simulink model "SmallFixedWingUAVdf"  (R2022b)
settings: Solver=ode4  StartTime=0  StopTime=stoptime  FixedStep=0.001  RelTol=1e-3  EnableMultiTasking=on
PreLoadFcn:
  | asbswarm_vehicledata; % load in workspace variables
PostLoadFcn:
  | open_system([gcs,'/MATLAB Animation Display/MATLAB',10,'Animation']);
InitFcn:
  | InitDatactrl
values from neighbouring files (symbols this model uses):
  env = struct    [InitDatactrl.m]
  F = Fattr + Frep    [APF.m]
  q = ix-1    [bspline_deboor.m]
  SenorSampleTime = 0.01    [InitDatactrl.m]
  sensors = struct    [InitDatactrl.m]
  uav = struct    [InitDatactrl.m]    (also in InitDatactrldf.m)
undefined symbols (not defined in the file or in its folder): Busy, Continuous, DiscIntNeverNeededParam, Dryden, Earth, Light, MIL, Newton, pa28, r, Raphson, sigbuilder_block, Wait, WGS84
libraries: simulink x37, aerolibactuator x10, sharedtransform x6, aerolibatmos2 x4, aerolibasang x4, aerolibwind2 x4, aerolibtransform2 x3, aerolibconvert2 x3, aerolibfltsims x2, shared6dof x2, aerolibnav x2, aerolibanimutils x1
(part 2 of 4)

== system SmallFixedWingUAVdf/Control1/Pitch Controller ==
  Pitch cmd : Inport
  Pitch act : Inport  Port=2
  pqr : Inport  Port=3
  Add1 : Sum  Inputs=+-
  Add6 : Sum  Inputs=+-
  Gain2 : Gain  Gain=-1
  PID_Pitch : Subsystem
  PID_PitchRate : Subsystem
  Selector : Selector  InputPortWidth=3  IndexOptions=Index vector (dialog)  Indices=2  OutputSizes=1
  elevatorCmd : Outport  VectorParamsAs1DForOutWhenUnconnected=off
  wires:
  PID_PitchRate/1(y) -> Gain2/1  "elevatorCmd"
  [reset] -> PID_PitchRate/2(reset_i)
  [reset] -> PID_Pitch/2(reset_i)
  Add1/1 -> PID_Pitch/1(e_theta)
  Add6/1 -> PID_PitchRate/1(x)
  Pitch act/1 -> Add1/2
  Gain2/1 -> elevatorCmd/1
  Selector/1 -> Add6/2  "q"
  PID_Pitch/1(qCmd) -> Add6/1
  pqr/1 -> Selector/1
  Pitch cmd/1 -> Add1/1

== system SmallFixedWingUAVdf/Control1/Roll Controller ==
  Roll cmd : Inport
  Roll act : Inport  Port=2
  pqr : Inport  Port=3
  Add2 : Sum  Inputs=+-
  Add3 : Sum  Inputs=+-
  PID_Roll : Subsystem
  PID_RollRate : Subsystem
  Selector1 : Selector  InputPortWidth=3  IndexOptions=Index vector (dialog)  Indices=1  OutputSizes=1
  aileronCmd : Outport  VectorParamsAs1DForOutWhenUnconnected=off
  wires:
  PID_RollRate/1(y) -> aileronCmd/1  "aileronCmd"
  Add2/1 -> PID_Roll/1(x)
  Add3/1 -> PID_RollRate/1(x)
  Selector1/1 -> Add3/2
  [reset] -> PID_RollRate/2(reset_i)
  [reset] -> PID_Roll/2(reset_i)
  pqr/1 -> Selector1/1
  Roll act/1 -> Add2/2
  PID_Roll/1(y) -> Add3/1
  Roll cmd/1 -> Add2/1

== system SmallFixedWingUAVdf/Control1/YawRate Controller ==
  psi_dot Cmd : Inport
  psi_dot : Inport  Port=2
  <YawRateCmd> : Inport  Port=3
  Add4 : Sum  Inputs=+-
  PID_YawRate : Subsystem
  Sum2 : Sum  Inputs=++|
  rudderCmd : Outport  VectorParamsAs1DForOutWhenUnconnected=off
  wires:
  Sum2/1 -> rudderCmd/1  "rudderCmd"
  Add4/1 -> PID_YawRate/1(x)
  [reset] -> PID_YawRate/2(reset_i)
  PID_YawRate/1(y) -> Sum2/2
  psi_dot/1 -> Add4/2
  psi_dot Cmd/1 -> Add4/1

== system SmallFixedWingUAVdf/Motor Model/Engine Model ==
  dt : Inport
  Airspeed : Inport  Port=2
  Constant4 : Constant  Value=0
  Get To : Subsystem
  Mass Conversion : aerolibconvert2/Mass Conversion  IU=lbm  OU=kg
  Mux : Mux  Inputs=2
  Mux1 : Mux  Inputs=3
  Thrust Available (lbs) : Fcn  Expr=u(1) - 0.047*sqrt(u(1))*u(2)
  kg2N : Gain  Gain=env.ISA_g  SaturateOnIntegerOverflow=on
  Thrust_b : Outport  Unit=kg*m/s^2  VectorParamsAs1DForOutWhenUnconnected=off
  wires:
  kg2N/1 -> Mux1/1
  Constant4/1 -> Mux1/3, Mux1/2
  Mass Conversion/1 -> kg2N/1
  Mux1/1 -> Thrust_b/1
  Airspeed/1 -> Mux/2
  Thrust Available (lbs)/1 -> Mass Conversion/1
  Mux/1 -> Thrust Available (lbs)/1
  Get To/1(To) -> Mux/1
  dt/1 -> Get To/1(dt)

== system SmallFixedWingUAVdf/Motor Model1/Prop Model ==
  dt : Inport
  Airspeed : Inport  Port=2
  Constant : Constant  Value=uav.prop.Ct
  Constant1 : Constant  Value=env.ISA_rho0
  Constant2 : Constant  Value=uav.prop.Dp
  Constant3 : Constant  Value=uav.prop.decay
  Constant4 : Constant  Value=0
  Constant5 : Constant  Value=uav.prop.Kv
  Constant6 : Constant  Value=uav.prop.U
  Mux : Mux  Inputs=3
  Mux1 : Mux  Inputs=3
  Product : Product  Inputs=4
  Product1 : Product  Inputs=3
  Saturation : Saturate  UpperLimit=1.0  LowerLimit=0
  Saturation1 : Saturate  UpperLimit=inf  LowerLimit=0
  Square : Math  Operator=square
  Square1 : Math  Operator=square
  Square2 : Math  Operator=square
  decay : Fcn  Expr=u(1)-u(3)*abs(u(2))/sqrt(u(1))
  min->s : Gain  Gain=1/60
  Thrust_b : Outport  Unit=kg*m/s^2  VectorParamsAs1DForOutWhenUnconnected=off
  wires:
  Constant4/1 -> Mux1/2, Mux1/3
  Product/1 -> Mux/1  "T0"
  Mux1/1 -> Thrust_b/1
  dt/1 -> Saturation/1
  Product1/1 -> min->s/1  "N"
  Airspeed/1 -> Mux/2  "Airspeed"
  Constant/1 -> Product/1
  min->s/1 -> Square/1
  Constant1/1 -> Product/2
  Constant2/1 -> Square2/1
  Square1/1 -> Product/3
  Square2/1 -> Square1/1
  Square/1 -> Product/4
  Saturation/1 -> Product1/1
  Mux/1 -> decay/1
  Constant3/1 -> Mux/3
  decay/1 -> Saturation1/1  "T"
  Saturation1/1 -> Mux1/1
  Constant5/1 -> Product1/2
  Constant6/1 -> Product1/3

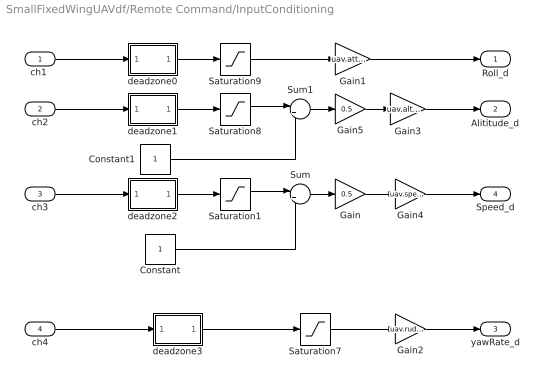
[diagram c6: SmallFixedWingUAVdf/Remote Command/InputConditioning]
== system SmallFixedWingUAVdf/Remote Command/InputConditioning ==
  "ch1 " : Inport
  ch2 : Inport  Port=2
  ch3 : Inport  Port=3
  ch4 : Inport  Port=4
  Constant : Constant
  Constant1 : Constant
  Gain : Gain  Gain=0.5
  Gain1 : Gain  Gain=uav.attitudectrlmax.roll  OutDataTypeStr=Inherit: Inherit via back propagation
  Gain2 : Gain  Gain=uav.rudder.max
  Gain3 : Gain  Gain=uav.altitude.max  OutDataTypeStr=Inherit: Inherit via back propagation
  Gain4 : Gain  Gain=uav.speed.max
  Gain5 : Gain  Gain=0.5
  Saturation{1,7..9} (4 alike) : Saturate  UpperLimit=1  LowerLimit=-1
  Sum : Sum  Inputs=|++
  Sum1 : Sum  Inputs=|++
  deadzone0 : MATLAB Function  TreatAsAtomicUnit=on
  deadzone1 : MATLAB Function  TreatAsAtomicUnit=on
  deadzone2 : MATLAB Function  TreatAsAtomicUnit=on
  deadzone3 : MATLAB Function  TreatAsAtomicUnit=on
  Roll_d : Outport  VectorParamsAs1DForOutWhenUnconnected=off
  Alititude_d : Outport  Port=2  VectorParamsAs1DForOutWhenUnconnected=off
  yawRate_d : Outport  Port=3  VectorParamsAs1DForOutWhenUnconnected=off
  Speed_d : Outport  Port=4  VectorParamsAs1DForOutWhenUnconnected=off
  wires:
  deadzone2/1(y) -> Saturation1/1
  ch3/1 -> deadzone2/1(u)
  deadzone1/1(y) -> Saturation8/1
  Gain/1 -> Gain4/1
  deadzone0/1(y) -> Saturation9/1
  "ch1 "/1 -> deadzone0/1(u)
  ch2/1 -> deadzone1/1(u)
  Saturation9/1 -> Gain1/1
  Constant/1 -> Sum/2
  Sum/1 -> Gain/1
  Gain1/1 -> Roll_d/1
  Gain3/1 -> Alititude_d/1
  Saturation7/1 -> Gain2/1
  deadzone3/1(y) -> Saturation7/1
  ch4/1 -> deadzone3/1(u)
  Gain2/1 -> yawRate_d/1
  Saturation1/1 -> Sum/1
  Gain4/1 -> Speed_d/1
  Sum1/1 -> Gain5/1
  Constant1/1 -> Sum1/2
  Saturation8/1 -> Sum1/1
  Gain5/1 -> Gain3/1

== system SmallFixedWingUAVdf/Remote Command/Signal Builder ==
  Demux : Demux  Tag=STV Demux  Outputs=1
  FromWs : FromWorkspace  Tag=STV FromWs  VariableName=tuvar
  Signal 1 : Outport  Tag=STV Outport  VectorParamsAs1DForOutWhenUnconnected=off
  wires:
  Demux/1 -> Signal 1/1
  FromWs/1 -> Demux/1

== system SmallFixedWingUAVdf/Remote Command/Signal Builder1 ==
  Demux : Demux  Tag=STV Demux  Outputs=1
  FromWs : FromWorkspace  Tag=STV FromWs  VariableName=tuvar
  Signal 1 : Outport  Tag=STV Outport  VectorParamsAs1DForOutWhenUnconnected=off
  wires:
  FromWs/1 -> Demux/1
  Demux/1 -> Signal 1/1

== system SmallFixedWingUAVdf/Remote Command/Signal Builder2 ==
  Demux : Demux  Tag=STV Demux  Outputs=1
  FromWs : FromWorkspace  Tag=STV FromWs  VariableName=tuvar
  Signal 1 : Outport  Tag=STV Outport  VectorParamsAs1DForOutWhenUnconnected=off
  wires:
  FromWs/1 -> Demux/1
  Demux/1 -> Signal 1/1

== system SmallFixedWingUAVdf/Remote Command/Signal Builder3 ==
  Demux : Demux  Tag=STV Demux  Outputs=1
  FromWs : FromWorkspace  Tag=STV FromWs  VariableName=tuvar
  Signal 1 : Outport  Tag=STV Outport  VectorParamsAs1DForOutWhenUnconnected=off
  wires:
  Demux/1 -> Signal 1/1
  FromWs/1 -> Demux/1

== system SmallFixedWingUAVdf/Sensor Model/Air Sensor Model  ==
  uavState : Inport
  AirData : Inport  Port=2
  Bus Creator : BusCreator  Inputs=4
  Bus Selector1 : BusSelector  OutputSignals=airpseed,q
  Bus Selector3 : BusSelector  OutputSignals=Xe
  Gain : Gain  Gain=-1
  Get Z : Selector  InputPortWidth=3  IndexOptions=Index vector (dialog)  Indices=[3]  OutputSizes=[(-2)]
  ISA Atmosphere Model : aerolibatmos2/ISA Atmosphere Model  custom=on  g=env.ISA_g  gamma=1.4  R=env.ISA_R  L=env.ISA_lapse  h_trop=11000  h_strat=20000  rho0=env.ISA_rho0  P0=env.ISA_P0  T0=env.ISA_T0  h0=0
  Temperature Conversion : aerolibconvert2/Temperature Conversion  IU=K  OU=C
  Terminator : Terminator
  Terminator1 : Terminator
  Transfer Fcn : TransferFcn  Denominator=[.01 1]
  AirSensorData : Outport  VectorParamsAs1DForOutWhenUnconnected=off
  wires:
  Bus Selector3/1 -> Get Z/1  "<Xe>"
  Get Z/1 -> Transfer Fcn/1
  Temperature Conversion/1 -> Bus Creator/1  "OAT"
  Bus Selector1/1 -> Bus Creator/3  "<airpseed>"
  Bus Selector1/2 -> Bus Creator/4  "<q>"
  ISA Atmosphere Model/1 -> Temperature Conversion/1  "OAT"
  Bus Creator/1 -> AirSensorData/1
  Gain/1 -> ISA Atmosphere Model/1
  ISA Atmosphere Model/3 -> Bus Creator/2  "static"
  ISA Atmosphere Model/2 -> Terminator1/1
  AirData/1 -> Bus Selector1/1
  Transfer Fcn/1 -> Gain/1
  uavState/1 -> Bus Selector3/1
  ISA Atmosphere Model/4 -> Terminator/1

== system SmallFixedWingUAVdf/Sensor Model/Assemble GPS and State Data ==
  UAVState : Inport
  AirSensorData : Inport  Port=2
  CtrlSurfaces : Inport  Port=3
  Bus Creator : BusCreator  Inputs=12
  Bus Selector : BusSelector  OutputSignals=static,q,OAT,airpseed
  Bus Selector1 : BusSelector  OutputSignals=dE,dA,dR,dF,dT
  Bus Selector2 : BusSelector  OutputSignals=Euler,pqr,Xe,Ve,Ab
  Bus Selector3 : BusSelector  OutputSignals=Xe
  Bus Selector4 : BusSelector  OutputSignals=gps_latLon,gps_h
  Generate GPS Data : Subsystem
  Mux : Mux  Inputs=5
  UAVStateBus : Outport  VectorParamsAs1DForOutWhenUnconnected=off
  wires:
  Mux/1 -> Bus Creator/12  "ctrlSurfacePos"
  Bus Selector1/5 -> Mux/5  "<dT>"
  Bus Selector1/4 -> Mux/4  "<dF>"
  Bus Selector1/3 -> Mux/3  "<dR>"
  Bus Selector1/2 -> Mux/2  "<dA>"
  Bus Selector1/1 -> Mux/1  "<dE>"
  CtrlSurfaces/1 -> Bus Selector1/1  "ctrlSurfacePos"
  Bus Selector4/2 -> Bus Creator/11  "<gps_h>"
  Bus Selector4/1 -> Bus Creator/10  "<gps_latLon>"
  Bus Selector/4 -> Bus Creator/9  "<airpseed>"
  Bus Selector/3 -> Bus Creator/8  "<OAT>"
  Bus Selector/2 -> Bus Creator/7  "<q>"
  Bus Selector/1 -> Bus Creator/6  "<static>"
  Bus Selector2/5 -> Bus Creator/5  "<Ab>"
  Bus Selector2/4 -> Bus Creator/4  "<Ve>"
  Bus Selector2/2 -> Bus Creator/2  "<pqr>"
  Bus Selector2/1 -> Bus Creator/1  "<Euler>"
  Generate GPS Data/1(GPSData) -> Bus Selector4/1
  Bus Creator/1 -> UAVStateBus/1
  UAVState/1 -> Bus Selector2/1, Bus Selector3/1
  Bus Selector3/1 -> Generate GPS Data/1(XYZ (NEU))  "<Xe>"
  AirSensorData/1 -> Bus Selector/1
  Bus Selector2/3 -> Bus Creator/3  "<Xe>"

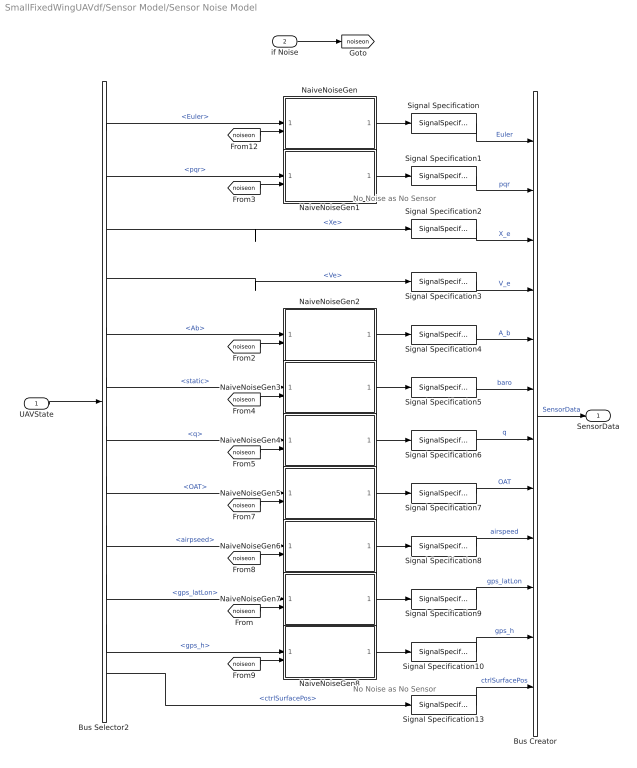
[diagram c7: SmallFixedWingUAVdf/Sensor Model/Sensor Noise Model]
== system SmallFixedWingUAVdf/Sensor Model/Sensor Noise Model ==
  note: No Noise as No Sensor
  note: No Noise as No Sensor
  UAVState : Inport
  if Noise : Inport  Port=2
  Bus Creator : BusCreator  Inputs=12
  Bus Selector2 : BusSelector  OutputSignals=Euler,pqr,Xe,Ve,Ab,static,q,OAT,airpseed,gps_latLon,gps_h,ctrlSurfacePos
  NaiveNoiseGen : Subsystem  mask{np=[0.0005 0.0005 0.0005], st=SenorSampleTime, ng=0.05, ns=[132 456 789]}
      mask prompts: np "Noise Power"; st "Sample Time"; ng "Noise Gain"; ns "Noise Seed"
  NaiveNoiseGen1 : Subsystem  mask{np=[0.0005 0.0005 0.0005], st=SenorSampleTime, ng=0.01, ns=[4132 4456 4789]}
      mask prompts: np "Noise Power"; st "Sample Time"; ng "Noise Gain"; ns "Noise Seed"
  NaiveNoiseGen2 : Subsystem  mask{np=[0.0005 0.0005 0.0005], st=SenorSampleTime, ng=0.01, ns=[138 458 788]}
      mask prompts: np "Noise Power"; st "Sample Time"; ng "Noise Gain"; ns "Noise Seed"
  NaiveNoiseGen3 : Subsystem  mask{np=[0.0005], st=SenorSampleTime, ng=0.2, ns=[1387]}
      mask prompts: np "Noise Power"; st "Sample Time"; ng "Noise Gain"; ns "Noise Seed"
  NaiveNoiseGen4 : Subsystem  mask{np=[0.0005], st=SenorSampleTime, ng=0.15, ns=[1317]}
      mask prompts: np "Noise Power"; st "Sample Time"; ng "Noise Gain"; ns "Noise Seed"
  NaiveNoiseGen5 : Subsystem  mask{np=[0.0005], st=SenorSampleTime, ng=0.2, ns=[1917]}
      mask prompts: np "Noise Power"; st "Sample Time"; ng "Noise Gain"; ns "Noise Seed"
  NaiveNoiseGen6 : Subsystem  mask{np=[0.0005], st=SenorSampleTime, ng=0.15, ns=[1557]}
      mask prompts: np "Noise Power"; st "Sample Time"; ng "Noise Gain"; ns "Noise Seed"
  NaiveNoiseGen7 : Subsystem  mask{np=[0.0001 0.0001], st=SenorSampleTime, ng=0.00001, ns=[138 458]}
      mask prompts: np "Noise Power"; st "Sample Time"; ng "Noise Gain"; ns "Noise Seed"
  NaiveNoiseGen8 : Subsystem  mask{np=[0.0005], st=SenorSampleTime, ng=0.15, ns=[7757]}
      mask prompts: np "Noise Power"; st "Sample Time"; ng "Noise Gain"; ns "Noise Seed"
  Signal Specification : SignalSpecification  Unit=rad
  Signal Specification1 : SignalSpecification  Unit=rad/s
  Signal Specification10 : SignalSpecification  Unit=m
  Signal Specification13 : SignalSpecification  Unit=rad
  Signal Specification2 : SignalSpecification  Unit=m
  Signal Specification3 : SignalSpecification  Unit=m/s
  Signal Specification4 : SignalSpecification  Unit=m/s^2
  Signal Specification5 : SignalSpecification  Unit=Pa
  Signal Specification6 : SignalSpecification  Unit=Pa
  Signal Specification7 : SignalSpecification  Unit=°C
  Signal Specification8 : SignalSpecification  Unit=m/s
  Signal Specification9 : SignalSpecification  Unit=deg
  SensorData : Outport  VectorParamsAs1DForOutWhenUnconnected=off
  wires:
  Bus Selector2/12 -> Signal Specification13/1  "<ctrlSurfacePos>"
  [noiseon] -> NaiveNoiseGen7/2(Noise On)
  Bus Selector2/10 -> NaiveNoiseGen7/1(Signal In)  "<gps_latLon>"
  Bus Selector2/11 -> NaiveNoiseGen8/1(Signal In)  "<gps_h>"
  [noiseon] -> NaiveNoiseGen8/2(Noise On)
  NaiveNoiseGen7/1(Signal Out) -> Signal Specification9/1
  Bus Creator/1 -> SensorData/1  "SensorData"
  NaiveNoiseGen8/1(Signal Out) -> Signal Specification10/1
  NaiveNoiseGen6/1(Signal Out) -> Signal Specification8/1
  NaiveNoiseGen5/1(Signal Out) -> Signal Specification7/1
  NaiveNoiseGen4/1(Signal Out) -> Signal Specification6/1
  NaiveNoiseGen3/1(Signal Out) -> Signal Specification5/1
  NaiveNoiseGen2/1(Signal Out) -> Signal Specification4/1
  NaiveNoiseGen1/1(Signal Out) -> Signal Specification1/1
  NaiveNoiseGen/1(Signal Out) -> Signal Specification/1
  Bus Selector2/9 -> NaiveNoiseGen6/1(Signal In)  "<airpseed>"
  Bus Selector2/8 -> NaiveNoiseGen5/1(Signal In)  "<OAT>"
  [noiseon] -> NaiveNoiseGen5/2(Noise On)
  [noiseon] -> NaiveNoiseGen6/2(Noise On)
  Bus Selector2/7 -> NaiveNoiseGen4/1(Signal In)  "<q>"
  Bus Selector2/2 -> NaiveNoiseGen1/1(Signal In)  "<pqr>"
  Bus Selector2/1 -> NaiveNoiseGen/1(Signal In)  "<Euler>"
  [noiseon] -> NaiveNoiseGen1/2(Noise On)
  if Noise/1 -> [noiseon]
  [noiseon] -> NaiveNoiseGen3/2(Noise On)
  [noiseon] -> NaiveNoiseGen4/2(Noise On)
  [noiseon] -> NaiveNoiseGen2/2(Noise On)
  [noiseon] -> NaiveNoiseGen/2(Noise On)
  UAVState/1 -> Bus Selector2/1
  Signal Specification/1 -> Bus Creator/1  "Euler"
  Signal Specification1/1 -> Bus Creator/2  "pqr"
  Signal Specification2/1 -> Bus Creator/3  "X_e"
  Signal Specification3/1 -> Bus Creator/4  "V_e"
  Signal Specification4/1 -> Bus Creator/5  "A_b"
  Signal Specification5/1 -> Bus Creator/6  "baro"
  Signal Specification6/1 -> Bus Creator/7  "q"
  Signal Specification7/1 -> Bus Creator/8  "OAT"
  Signal Specification8/1 -> Bus Creator/9  "airspeed"
  Signal Specification9/1 -> Bus Creator/10  "gps_latLon"
  Signal Specification10/1 -> Bus Creator/11  "gps_h"
  Signal Specification13/1 -> Bus Creator/12  "ctrlSurfacePos"
  Bus Selector2/6 -> NaiveNoiseGen3/1(Signal In)  "<static>"
  Bus Selector2/5 -> NaiveNoiseGen2/1(Signal In)  "<Ab>"
  Bus Selector2/3 -> Signal Specification2/1  "<Xe>"
  Bus Selector2/4 -> Signal Specification3/1  "<Ve>"

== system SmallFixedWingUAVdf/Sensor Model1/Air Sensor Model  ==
  uavState : Inport
  AirData : Inport  Port=2
  Bus Creator : BusCreator  Inputs=4
  Bus Selector1 : BusSelector  OutputSignals=airpseed,q
  Bus Selector3 : BusSelector  OutputSignals=Xe
  Gain : Gain  Gain=-1
  Get Z : Selector  InputPortWidth=3  IndexOptions=Index vector (dialog)  Indices=[3]  OutputSizes=[(-2)]
  ISA Atmosphere Model : aerolibatmos2/ISA Atmosphere Model  custom=on  g=env.ISA_g  gamma=1.4  R=env.ISA_R  L=env.ISA_lapse  h_trop=11000  h_strat=20000  rho0=env.ISA_rho0  P0=env.ISA_P0  T0=env.ISA_T0  h0=0
  Temperature Conversion : aerolibconvert2/Temperature Conversion  IU=K  OU=C
  Terminator : Terminator
  Terminator1 : Terminator
  Transfer Fcn : TransferFcn  Denominator=[.01 1]
  AirSensorData : Outport  VectorParamsAs1DForOutWhenUnconnected=off
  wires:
  Bus Selector3/1 -> Get Z/1  "<Xe>"
  Get Z/1 -> Transfer Fcn/1
  Temperature Conversion/1 -> Bus Creator/1  "OAT"
  Bus Selector1/1 -> Bus Creator/3  "<airpseed>"
  Bus Selector1/2 -> Bus Creator/4  "<q>"
  ISA Atmosphere Model/1 -> Temperature Conversion/1  "OAT"
  Bus Creator/1 -> AirSensorData/1
  Gain/1 -> ISA Atmosphere Model/1
  ISA Atmosphere Model/3 -> Bus Creator/2  "static"
  ISA Atmosphere Model/2 -> Terminator1/1
  AirData/1 -> Bus Selector1/1
  Transfer Fcn/1 -> Gain/1
  uavState/1 -> Bus Selector3/1
  ISA Atmosphere Model/4 -> Terminator/1

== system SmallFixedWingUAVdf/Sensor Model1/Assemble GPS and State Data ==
  UAVState : Inport
  AirSensorData : Inport  Port=2
  CtrlSurfaces : Inport  Port=3
  Bus Creator : BusCreator  Inputs=12
  Bus Selector : BusSelector  OutputSignals=static,q,OAT,airpseed
  Bus Selector1 : BusSelector  OutputSignals=dE,dA,dR,dF,dT
  Bus Selector2 : BusSelector  OutputSignals=Euler,pqr,Xe,Ve,Ab
  Bus Selector3 : BusSelector  OutputSignals=Xe
  Bus Selector4 : BusSelector  OutputSignals=gps_latLon,gps_h
  Generate GPS Data : Subsystem
  Mux : Mux  Inputs=5
  UAVStateBus : Outport  VectorParamsAs1DForOutWhenUnconnected=off
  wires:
  Mux/1 -> Bus Creator/12  "ctrlSurfacePos"
  Bus Selector1/5 -> Mux/5  "<dT>"
  Bus Selector1/4 -> Mux/4  "<dF>"
  Bus Selector1/3 -> Mux/3  "<dR>"
  Bus Selector1/2 -> Mux/2  "<dA>"
  Bus Selector1/1 -> Mux/1  "<dE>"
  CtrlSurfaces/1 -> Bus Selector1/1  "ctrlSurfacePos"
  Bus Selector4/2 -> Bus Creator/11  "<gps_h>"
  Bus Selector4/1 -> Bus Creator/10  "<gps_latLon>"
  Bus Selector/4 -> Bus Creator/9  "<airpseed>"
  Bus Selector/3 -> Bus Creator/8  "<OAT>"
  Bus Selector/2 -> Bus Creator/7  "<q>"
  Bus Selector/1 -> Bus Creator/6  "<static>"
  Bus Selector2/5 -> Bus Creator/5  "<Ab>"
  Bus Selector2/4 -> Bus Creator/4  "<Ve>"
  Bus Selector2/2 -> Bus Creator/2  "<pqr>"
  Bus Selector2/1 -> Bus Creator/1  "<Euler>"
  Generate GPS Data/1(GPSData) -> Bus Selector4/1
  Bus Creator/1 -> UAVStateBus/1
  UAVState/1 -> Bus Selector2/1, Bus Selector3/1
  Bus Selector3/1 -> Generate GPS Data/1(XYZ (NEU))  "<Xe>"
  AirSensorData/1 -> Bus Selector/1
  Bus Selector2/3 -> Bus Creator/3  "<Xe>"

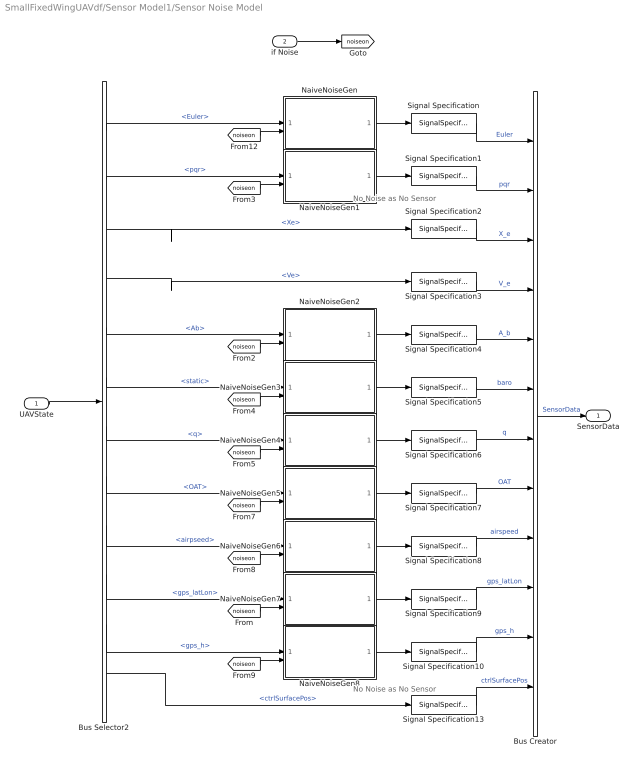
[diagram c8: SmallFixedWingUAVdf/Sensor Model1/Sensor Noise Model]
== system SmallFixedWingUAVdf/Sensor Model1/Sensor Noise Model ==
  note: No Noise as No Sensor
  note: No Noise as No Sensor
  UAVState : Inport
  if Noise : Inport  Port=2
  Bus Creator : BusCreator  Inputs=12
  Bus Selector2 : BusSelector  OutputSignals=Euler,pqr,Xe,Ve,Ab,static,q,OAT,airpseed,gps_latLon,gps_h,ctrlSurfacePos
  NaiveNoiseGen : Subsystem  mask{np=[0.0005 0.0005 0.0005], st=SenorSampleTime, ng=0.05, ns=[132 456 789]}
      mask prompts: np "Noise Power"; st "Sample Time"; ng "Noise Gain"; ns "Noise Seed"
  NaiveNoiseGen1 : Subsystem  mask{np=[0.0005 0.0005 0.0005], st=SenorSampleTime, ng=0.01, ns=[4132 4456 4789]}
      mask prompts: np "Noise Power"; st "Sample Time"; ng "Noise Gain"; ns "Noise Seed"
  NaiveNoiseGen2 : Subsystem  mask{np=[0.0005 0.0005 0.0005], st=SenorSampleTime, ng=0.01, ns=[138 458 788]}
      mask prompts: np "Noise Power"; st "Sample Time"; ng "Noise Gain"; ns "Noise Seed"
  NaiveNoiseGen3 : Subsystem  mask{np=[0.0005], st=SenorSampleTime, ng=0.2, ns=[1387]}
      mask prompts: np "Noise Power"; st "Sample Time"; ng "Noise Gain"; ns "Noise Seed"
  NaiveNoiseGen4 : Subsystem  mask{np=[0.0005], st=SenorSampleTime, ng=0.15, ns=[1317]}
      mask prompts: np "Noise Power"; st "Sample Time"; ng "Noise Gain"; ns "Noise Seed"
  NaiveNoiseGen5 : Subsystem  mask{np=[0.0005], st=SenorSampleTime, ng=0.2, ns=[1917]}
      mask prompts: np "Noise Power"; st "Sample Time"; ng "Noise Gain"; ns "Noise Seed"
  NaiveNoiseGen6 : Subsystem  mask{np=[0.0005], st=SenorSampleTime, ng=0.15, ns=[1557]}
      mask prompts: np "Noise Power"; st "Sample Time"; ng "Noise Gain"; ns "Noise Seed"
  NaiveNoiseGen7 : Subsystem  mask{np=[0.0001 0.0001], st=SenorSampleTime, ng=0.00001, ns=[138 458]}
      mask prompts: np "Noise Power"; st "Sample Time"; ng "Noise Gain"; ns "Noise Seed"
  NaiveNoiseGen8 : Subsystem  mask{np=[0.0005], st=SenorSampleTime, ng=0.15, ns=[7757]}
      mask prompts: np "Noise Power"; st "Sample Time"; ng "Noise Gain"; ns "Noise Seed"
  Signal Specification : SignalSpecification  Unit=rad
  Signal Specification1 : SignalSpecification  Unit=rad/s
  Signal Specification10 : SignalSpecification  Unit=m
  Signal Specification13 : SignalSpecification  Unit=rad
  Signal Specification2 : SignalSpecification  Unit=m
  Signal Specification3 : SignalSpecification  Unit=m/s
  Signal Specification4 : SignalSpecification  Unit=m/s^2
  Signal Specification5 : SignalSpecification  Unit=Pa
  Signal Specification6 : SignalSpecification  Unit=Pa
  Signal Specification7 : SignalSpecification  Unit=°C
  Signal Specification8 : SignalSpecification  Unit=m/s
  Signal Specification9 : SignalSpecification  Unit=deg
  SensorData : Outport  VectorParamsAs1DForOutWhenUnconnected=off
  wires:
  Bus Selector2/12 -> Signal Specification13/1  "<ctrlSurfacePos>"
  [noiseon] -> NaiveNoiseGen7/2(Noise On)
  Bus Selector2/10 -> NaiveNoiseGen7/1(Signal In)  "<gps_latLon>"
  Bus Selector2/11 -> NaiveNoiseGen8/1(Signal In)  "<gps_h>"
  [noiseon] -> NaiveNoiseGen8/2(Noise On)
  NaiveNoiseGen7/1(Signal Out) -> Signal Specification9/1
  Bus Creator/1 -> SensorData/1  "SensorData"
  NaiveNoiseGen8/1(Signal Out) -> Signal Specification10/1
  NaiveNoiseGen6/1(Signal Out) -> Signal Specification8/1
  NaiveNoiseGen5/1(Signal Out) -> Signal Specification7/1
  NaiveNoiseGen4/1(Signal Out) -> Signal Specification6/1
  NaiveNoiseGen3/1(Signal Out) -> Signal Specification5/1
  NaiveNoiseGen2/1(Signal Out) -> Signal Specification4/1
  NaiveNoiseGen1/1(Signal Out) -> Signal Specification1/1
  NaiveNoiseGen/1(Signal Out) -> Signal Specification/1
  Bus Selector2/9 -> NaiveNoiseGen6/1(Signal In)  "<airpseed>"
  Bus Selector2/8 -> NaiveNoiseGen5/1(Signal In)  "<OAT>"
  [noiseon] -> NaiveNoiseGen5/2(Noise On)
  [noiseon] -> NaiveNoiseGen6/2(Noise On)
  Bus Selector2/7 -> NaiveNoiseGen4/1(Signal In)  "<q>"
  Bus Selector2/4 -> Signal Specification3/1  "<Ve>"
  Bus Selector2/3 -> Signal Specification2/1  "<Xe>"
  Bus Selector2/2 -> NaiveNoiseGen1/1(Signal In)  "<pqr>"
  Bus Selector2/1 -> NaiveNoiseGen/1(Signal In)  "<Euler>"
  [noiseon] -> NaiveNoiseGen1/2(Noise On)
  if Noise/1 -> [noiseon]
  [noiseon] -> NaiveNoiseGen3/2(Noise On)
  [noiseon] -> NaiveNoiseGen4/2(Noise On)
  [noiseon] -> NaiveNoiseGen2/2(Noise On)
  [noiseon] -> NaiveNoiseGen/2(Noise On)
  UAVState/1 -> Bus Selector2/1
  Signal Specification/1 -> Bus Creator/1  "Euler"
  Signal Specification1/1 -> Bus Creator/2  "pqr"
  Signal Specification2/1 -> Bus Creator/3  "X_e"
  Signal Specification3/1 -> Bus Creator/4  "V_e"
  Signal Specification4/1 -> Bus Creator/5  "A_b"
  Signal Specification5/1 -> Bus Creator/6  "baro"
  Signal Specification6/1 -> Bus Creator/7  "q"
  Signal Specification7/1 -> Bus Creator/8  "OAT"
  Signal Specification8/1 -> Bus Creator/9  "airspeed"
  Signal Specification9/1 -> Bus Creator/10  "gps_latLon"
  Signal Specification10/1 -> Bus Creator/11  "gps_h"
  Signal Specification13/1 -> Bus Creator/12  "ctrlSurfacePos"
  Bus Selector2/6 -> NaiveNoiseGen3/1(Signal In)  "<static>"
  Bus Selector2/5 -> NaiveNoiseGen2/1(Signal In)  "<Ab>"

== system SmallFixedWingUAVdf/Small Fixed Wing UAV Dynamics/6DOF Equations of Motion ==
  FM_b : Inport
  6DOF (Euler Angles) : shared6dof/6DOF (Euler Angles)  units=Metric (MKS)  mtype=Fixed  rep=Euler Angles  xme_0=uav.ic.Pos_0.*double([1; 1; -1])  Vm_0=uav.ic.Vb_0  eul_0=uav.ic.Euler_0  pm_0=uav.ic.PQR_0  mass_0=uav.geometry.mass  mass_e=0.5  mass_f=2.0  inertia=eye(3).*[uav.inertia.Ixx;uav.inertia.Iyy; uav.inertia.Izz]  inertia_e=eye(3)  inertia_f=2*eye(3)  k_quat=1.0  vre_flag=on  abi_flag=off  aMode=0  xme_statename=''  Vm_statename=''  eul_statename=''  quat_statename=''  pm_statename=''  mass_statename=''
  Bus Creator : BusCreator  Inputs=8
  Compute psi_dot : Subsystem
  Constant : Constant  Value=[0 0 0]
  Demux2 : Demux  Outputs=2
  Three-axis Accelerometer : aerolibnav/Three-axis Accelerometer  units=Metric (MKS)  acc=[0 0 0]  gtype=off  dtype_a=off  w_a=190  z_a=0.707  a_sf_cc=[1 0 0; 0 1 0; 0 0 1]  a_bias=[0 0 0]  a_Ts=0  a_rand=off  a_seeds=[23093 23094 23095]  a_pow=[0.001 0.001 0.001]  a_sat="[-inf  -inf  -inf  inf inf inf]"
  "[0, pi] Wrap Around" : Subsystem
  UAVState : Outport  VectorParamsAs1DForOutWhenUnconnected=off
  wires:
  6DOF (Euler Angles)/7 -> Three-axis Accelerometer/3
  6DOF (Euler Angles)/6 -> Three-axis Accelerometer/2, Compute psi_dot/2(G), Bus Creator/6  "pqr"
  6DOF (Euler Angles)/2 -> Bus Creator/2  "Xe"
  6DOF (Euler Angles)/5 -> Bus Creator/5  "Vb"
  6DOF (Euler Angles)/4 -> Bus Creator/4  "DCM"
  Compute psi_dot/1(psi_dot) -> Bus Creator/7  "psi_dot"
  6DOF (Euler Angles)/1 -> Bus Creator/1  "Ve"
  6DOF (Euler Angles)/3 -> "[0, pi] Wrap Around"/1(Euler), Compute psi_dot/1(Euler)
  "[0, pi] Wrap Around"/1(Wrapped) -> Bus Creator/3  "Euler"
  6DOF (Euler Angles)/8 -> Three-axis Accelerometer/1
  Three-axis Accelerometer/1 -> Bus Creator/8  "Ab"
  Bus Creator/1 -> UAVState/1  "UAVState"
  Constant/1 -> Three-axis Accelerometer/4
  Demux2/1 -> 6DOF (Euler Angles)/1
  Demux2/2 -> 6DOF (Euler Angles)/2
  FM_b/1 -> Demux2/1

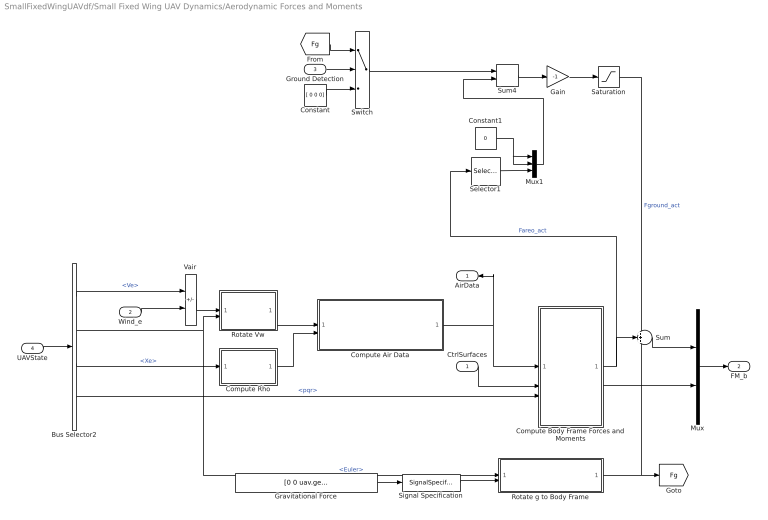
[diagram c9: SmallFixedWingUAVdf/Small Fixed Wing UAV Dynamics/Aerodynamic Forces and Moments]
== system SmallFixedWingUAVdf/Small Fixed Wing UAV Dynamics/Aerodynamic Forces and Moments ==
  CtrlSurfaces : Inport
  Wind_e : Inport  Port=2
  Ground Detection : Inport  Port=3
  UAVState : Inport  Port=4
  Bus Selector2 : BusSelector  OutputSignals=Ve,Euler,Xe,pqr
  Compute Air Data : Subsystem  TreatAsAtomicUnit=on  VariantControl=use_aerospace_blocks == 1
  Compute Body Frame Forces and Moments : Subsystem
  Compute Rho : Subsystem
  Constant : Constant  Value=[ 0 0 0]
  Constant1 : Constant  Value=0
  Gain : Gain  Gain=-1
  Gravitational Force : Constant  Value=[0 0 uav.geometry.mass*env.ISA_g]  VectorParams1D=off
  Mux : Mux  Inputs=2
  Mux1 : Mux  Inputs=3
  Rotate Vw : Subsystem
  Rotate g to Body Frame : Subsystem
  Saturation : Saturate  UpperLimit=0  LowerLimit=-inf
  Selector1 : Selector  InputPortWidth=3  IndexOptions=Index vector (dialog)  Indices=3  OutputSizes=1
  Signal Specification : SignalSpecification  Unit=kg*m/s^2
  Sum : Sum  Inputs=+++  SaturateOnIntegerOverflow=on
  Sum4 : Sum  InputSameDT=on  SaturateOnIntegerOverflow=on
  Switch : Switch  Criteria=u2 > Threshold  Threshold=0.3
  Vair : Sum  Inputs=+-  InputSameDT=on  SaturateOnIntegerOverflow=on
  AirData : Outport  VectorParamsAs1DForOutWhenUnconnected=off
  FM_b : Outport  Port=2  VectorParamsAs1DForOutWhenUnconnected=off
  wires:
  Bus Selector2/1 -> Vair/1  "<Ve>"
  UAVState/1 -> Bus Selector2/1
  Mux/1 -> FM_b/1
  Sum/1 -> Mux/1
  Wind_e/1 -> Vair/2
  CtrlSurfaces/1 -> Compute Body Frame Forces and Moments/2(CtrlSurfaces)
  Compute Air Data/1(AirData) -> AirData/1, Compute Body Frame Forces and Moments/1(AirData)
  Bus Selector2/4 -> Compute Body Frame Forces and Moments/3(p,q,r)  "<pqr>"
  Gravitational Force/1 -> Signal Specification/1
  Compute Body Frame Forces and Moments/2(M_b) -> Mux/2
  Rotate Vw/1(Vb) -> Compute Air Data/1(Vb)
  Compute Rho/1(Rho) -> Compute Air Data/2(Rho)
  Bus Selector2/2 -> Rotate g to Body Frame/1(Euler), Rotate Vw/2(Euler)  "<Euler>"
  Vair/1 -> Rotate Vw/1(Vw)
  Signal Specification/1 -> Rotate g to Body Frame/2(Gravity Force)
  Bus Selector2/3 -> Compute Rho/1(Xe)  "<Xe>"
  Saturation/1 -> Sum/1  "Fground_act"
  Gain/1 -> Saturation/1
  Switch/1 -> Sum4/1
  Constant1/1 -> Mux1/2, Mux1/1
  Mux1/1 -> Sum4/2
  Selector1/1 -> Mux1/3
  [Fg] -> Switch/1
  Sum4/1 -> Gain/1
  Compute Body Frame Forces and Moments/1(F_b) -> Sum/2, Selector1/1  "Fareo_act"
  Rotate g to Body Frame/1(g_b) -> [Fg], Sum/3
  Ground Detection/1 -> Switch/2
  Constant/1 -> Switch/3

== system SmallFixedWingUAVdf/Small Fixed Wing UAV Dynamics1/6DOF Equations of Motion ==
  FM_b : Inport
  6DOF (Euler Angles) : shared6dof/6DOF (Euler Angles)  units=Metric (MKS)  mtype=Fixed  rep=Euler Angles  xme_0=uav.ic.Pos_0.*[1; 1; -1]  Vm_0=uav.ic.Vb_0  eul_0=uav.ic.Euler_0  pm_0=uav.ic.PQR_0  mass_0=uav.geometry.mass  mass_e=0.5  mass_f=2.0  inertia="[uav.inertia.Ixx 0 -uav.inertia.Ixz;0 uav.inertia.Iyy 0;-uav.inertia.Ixz 0  uav.inertia.Izz]"  inertia_e=eye(3)  inertia_f=2*eye(3)  k_quat=1.0  vre_flag=on  abi_flag=off  aMode=0  xme_statename=''  Vm_statename=''  eul_statename=''  quat_statename=''  pm_statename=''  mass_statename=''
  Bus Creator : BusCreator  Inputs=8
  Compute psi_dot : Subsystem
  Constant : Constant  Value=[0 0 0]
  Demux2 : Demux  Outputs=2
  Three-axis Accelerometer : aerolibnav/Three-axis Accelerometer  units=Metric (MKS)  acc=[0 0 0]  gtype=off  dtype_a=off  w_a=190  z_a=0.707  a_sf_cc=[1 0 0; 0 1 0; 0 0 1]  a_bias=[0 0 0]  a_Ts=0  a_rand=off  a_seeds=[23093 23094 23095]  a_pow=[0.001 0.001 0.001]  a_sat="[-inf  -inf  -inf  inf inf inf]"
  "[0, pi] Wrap Around" : Subsystem
  UAVState : Outport  VectorParamsAs1DForOutWhenUnconnected=off
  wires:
  6DOF (Euler Angles)/7 -> Three-axis Accelerometer/3
  6DOF (Euler Angles)/6 -> Three-axis Accelerometer/2, Compute psi_dot/2(G), Bus Creator/6  "pqr"
  6DOF (Euler Angles)/2 -> Bus Creator/2  "Xe"
  6DOF (Euler Angles)/5 -> Bus Creator/5  "Vb"
  6DOF (Euler Angles)/4 -> Bus Creator/4  "DCM"
  Compute psi_dot/1(psi_dot) -> Bus Creator/7  "psi_dot"
  6DOF (Euler Angles)/1 -> Bus Creator/1  "Ve"
  6DOF (Euler Angles)/3 -> "[0, pi] Wrap Around"/1(Euler), Compute psi_dot/1(Euler)
  "[0, pi] Wrap Around"/1(Wrapped) -> Bus Creator/3  "Euler"
  6DOF (Euler Angles)/8 -> Three-axis Accelerometer/1
  Three-axis Accelerometer/1 -> Bus Creator/8  "Ab"
  Bus Creator/1 -> UAVState/1  "UAVState"
  Constant/1 -> Three-axis Accelerometer/4
  Demux2/1 -> 6DOF (Euler Angles)/1
  Demux2/2 -> 6DOF (Euler Angles)/2
  FM_b/1 -> Demux2/1

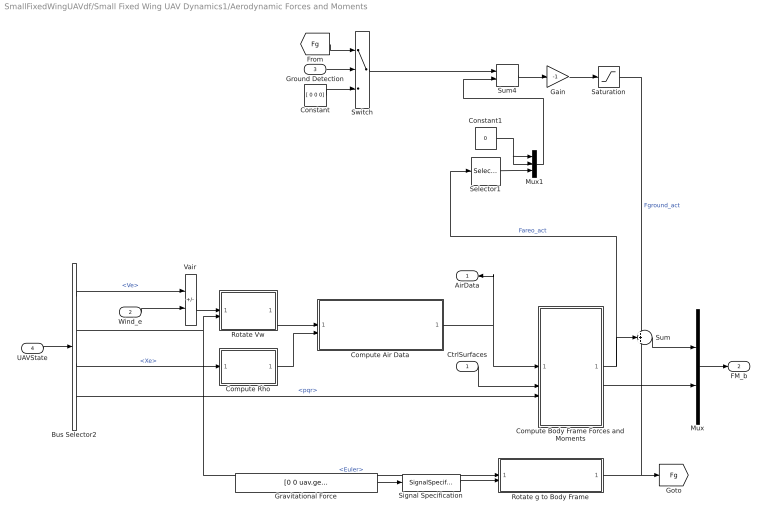
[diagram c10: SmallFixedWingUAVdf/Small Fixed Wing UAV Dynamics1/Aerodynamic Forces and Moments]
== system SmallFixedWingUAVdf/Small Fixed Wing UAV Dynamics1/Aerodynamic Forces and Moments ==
  CtrlSurfaces : Inport
  Wind_e : Inport  Port=2
  Ground Detection : Inport  Port=3
  UAVState : Inport  Port=4
  Bus Selector2 : BusSelector  OutputSignals=Ve,Euler,Xe,pqr
  Compute Air Data : Subsystem  TreatAsAtomicUnit=on  VariantControl=use_aerospace_blocks == 1
  Compute Body Frame Forces and Moments : Subsystem
  Compute Rho : Subsystem
  Constant : Constant  Value=[ 0 0 0]
  Constant1 : Constant  Value=0
  Gain : Gain  Gain=-1
  Gravitational Force : Constant  Value=[0 0 uav.geometry.mass*env.ISA_g]  VectorParams1D=off
  Mux : Mux  Inputs=2
  Mux1 : Mux  Inputs=3
  Rotate Vw : Subsystem
  Rotate g to Body Frame : Subsystem
  Saturation : Saturate  UpperLimit=0  LowerLimit=-inf
  Selector1 : Selector  InputPortWidth=3  IndexOptions=Index vector (dialog)  Indices=3  OutputSizes=1
  Signal Specification : SignalSpecification  Unit=kg*m/s^2
  Sum : Sum  Inputs=+++  SaturateOnIntegerOverflow=on
  Sum4 : Sum  InputSameDT=on  SaturateOnIntegerOverflow=on
  Switch : Switch  Criteria=u2 > Threshold  Threshold=0.3
  Vair : Sum  Inputs=+-  InputSameDT=on  SaturateOnIntegerOverflow=on
  AirData : Outport  VectorParamsAs1DForOutWhenUnconnected=off
  FM_b : Outport  Port=2  VectorParamsAs1DForOutWhenUnconnected=off
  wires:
  Bus Selector2/1 -> Vair/1  "<Ve>"
  UAVState/1 -> Bus Selector2/1
  Mux/1 -> FM_b/1
  Sum/1 -> Mux/1
  Wind_e/1 -> Vair/2
  CtrlSurfaces/1 -> Compute Body Frame Forces and Moments/2(CtrlSurfaces)
  Compute Air Data/1(AirData) -> AirData/1, Compute Body Frame Forces and Moments/1(AirData)
  Bus Selector2/4 -> Compute Body Frame Forces and Moments/3(p,q,r)  "<pqr>"
  Gravitational Force/1 -> Signal Specification/1
  Compute Body Frame Forces and Moments/2(M_b) -> Mux/2
  Rotate Vw/1(Vb) -> Compute Air Data/1(Vb)
  Compute Rho/1(Rho) -> Compute Air Data/2(Rho)
  Bus Selector2/2 -> Rotate g to Body Frame/1(Euler), Rotate Vw/2(Euler)  "<Euler>"
  Vair/1 -> Rotate Vw/1(Vw)
  Signal Specification/1 -> Rotate g to Body Frame/2(Gravity Force)
  Bus Selector2/3 -> Compute Rho/1(Xe)  "<Xe>"
  Saturation/1 -> Sum/1  "Fground_act"
  Gain/1 -> Saturation/1
  Switch/1 -> Sum4/1
  Constant1/1 -> Mux1/2, Mux1/1
  Mux1/1 -> Sum4/2
  Selector1/1 -> Mux1/3
  [Fg] -> Switch/1
  Sum4/1 -> Gain/1
  Compute Body Frame Forces and Moments/1(F_b) -> Sum/2, Selector1/1  "Fareo_act"
  Rotate g to Body Frame/1(g_b) -> [Fg], Sum/3
  Ground Detection/1 -> Switch/2
  Constant/1 -> Switch/3

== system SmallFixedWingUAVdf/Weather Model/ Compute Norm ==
  <Ve> : Inport
  Dot Product : DotProduct
  Math Function1 : Sqrt  AlgorithmType=Newton-Raphson
  Zero Bound : Saturate  UpperLimit=inf  LowerLimit=0.001
  V : Outport  VectorParamsAs1DForOutWhenUnconnected=off
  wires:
  Dot Product/1 -> Zero Bound/1
  Zero Bound/1 -> Math Function1/1
  <Ve>/1 -> Dot Product/2, Dot Product/1
  Math Function1/1 -> V/1

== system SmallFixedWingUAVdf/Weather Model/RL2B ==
  Euler : Inport
  Rotation Angles to Direction Cosine Matrix : sharedtransform/Rotation Angles to Direction Cosine Matrix  rotationOrder=ZYX  aMode=aMode
  Selector : Selector  InputPortWidth=3  IndexOptions=Index vector (dialog)  Indices=[3 2 1]  OutputSizes=1
  RL2B : Outport  VectorParamsAs1DForOutWhenUnconnected=off
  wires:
  Rotation Angles to Direction Cosine Matrix/1 -> RL2B/1
  Euler/1 -> Selector/1
  Selector/1 -> Rotation Angles to Direction Cosine Matrix/1

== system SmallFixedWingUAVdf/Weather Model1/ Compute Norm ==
  <Ve> : Inport
  Dot Product : DotProduct
  Math Function1 : Sqrt  AlgorithmType=Newton-Raphson
  Zero Bound : Saturate  UpperLimit=inf  LowerLimit=0.001
  V : Outport  VectorParamsAs1DForOutWhenUnconnected=off
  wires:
  Dot Product/1 -> Zero Bound/1
  Zero Bound/1 -> Math Function1/1
  <Ve>/1 -> Dot Product/2, Dot Product/1
  Math Function1/1 -> V/1

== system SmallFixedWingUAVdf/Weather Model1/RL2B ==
  Euler : Inport
  Rotation Angles to Direction Cosine Matrix : sharedtransform/Rotation Angles to Direction Cosine Matrix  rotationOrder=ZYX  aMode=aMode
  Selector : Selector  InputPortWidth=3  IndexOptions=Index vector (dialog)  Indices=[3 2 1]  OutputSizes=1
  RL2B : Outport  VectorParamsAs1DForOutWhenUnconnected=off
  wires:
  Rotation Angles to Direction Cosine Matrix/1 -> RL2B/1
  Euler/1 -> Selector/1
  Selector/1 -> Rotation Angles to Direction Cosine Matrix/1

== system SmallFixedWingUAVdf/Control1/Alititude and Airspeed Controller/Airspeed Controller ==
  Speed cmd : Inport
  speed act : Inport  Port=2
  Add7 : Sum  Inputs=+-
  PID_Speed : Subsystem
  y : Outport
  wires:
  [reset] -> PID_Speed/2(reset_i)
  PID_Speed/1(y) -> y/1
  Add7/1 -> PID_Speed/1(x)  "speederror"
  speed act/1 -> Add7/2
  Speed cmd/1 -> Add7/1

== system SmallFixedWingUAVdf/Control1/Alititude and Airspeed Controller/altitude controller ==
  Alititude cmd : Inport
  Alititude act : Inport  Port=2
  Add8 : Sum  Inputs=+-
  PID_Altitude : Subsystem
  pitchout : Outport
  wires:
  [reset] -> PID_Altitude/2(reset_i)
  PID_Altitude/1(y) -> pitchout/1  "pitchout"
  Add8/1 -> PID_Altitude/1(x)
  Alititude act/1 -> Add8/2
  Alititude cmd/1 -> Add8/1

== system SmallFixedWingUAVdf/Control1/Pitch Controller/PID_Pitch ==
  e_theta : Inport
  reset_i : Inport  Port=2
  Derivative Gain : Gain  DisableCoverage=on  Gain=0  ParamMin=-100  ParamMax=100  OutMin=-100  OutMax=100
  Discrete Derivative : simulink/Discrete/Discrete Derivative  gainval=1.0  ICPrevScaledInput=0.0  OutMin=[]  OutMax=[]  OutDataType=fixdt(1, 16)  OutScaling=2^-10  DoSatur=off
  Discrete-Time Integrator : DiscreteIntegrator  ExternalReset=either  SampleTime=-1  ICPrevOutput=DiscIntNeverNeededParam  ICPrevScaledInput=DiscIntNeverNeededParam
  Gain : Gain  Gain=6
  Integral Gain : Gain  DisableCoverage=on  Gain=0.4
  Sum : Sum  Inputs=+++
  qCmd : Outport  InitialOutput=0  VectorParamsAs1DForOutWhenUnconnected=off
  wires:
  e_theta/1 -> Gain/1, Integral Gain/1, Derivative Gain/1
  Integral Gain/1 -> Discrete-Time Integrator/1
  Derivative Gain/1 -> Discrete Derivative/1
  Gain/1 -> Sum/1
  Sum/1 -> qCmd/1
  Discrete Derivative/1 -> Sum/3
  Discrete-Time Integrator/1 -> Sum/2
  reset_i/1 -> Discrete-Time Integrator/2

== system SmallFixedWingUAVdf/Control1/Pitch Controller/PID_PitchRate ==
  x : Inport
  reset_i : Inport  Port=2
  Derivative Gain : Gain  DisableCoverage=on  Gain=0.04  ParamMin=-100  ParamMax=100  OutMin=-100  OutMax=100
  Discrete Derivative : simulink/Discrete/Discrete Derivative  gainval=1.0  ICPrevScaledInput=0.0  OutMin=[]  OutMax=[]  OutDataType=fixdt(1, 16)  OutScaling=2^-10  DoSatur=off
  Discrete-Time Integrator : DiscreteIntegrator  ExternalReset=either  SampleTime=-1  LimitOutput=on  UpperSaturationLimit=0.3  LowerSaturationLimit=-0.3  ICPrevOutput=DiscIntNeverNeededParam  ICPrevScaledInput=DiscIntNeverNeededParam
  Gain : Gain  Gain=0.8
  Integral Gain : Gain  DisableCoverage=on  Gain=12
  Sum : Sum  Inputs=+++
  y : Outport  InitialOutput=0  VectorParamsAs1DForOutWhenUnconnected=off
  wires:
  reset_i/1 -> Discrete-Time Integrator/2
  Discrete-Time Integrator/1 -> Sum/2
  Discrete Derivative/1 -> Sum/3
  Sum/1 -> y/1
  Gain/1 -> Sum/1
  Derivative Gain/1 -> Discrete Derivative/1
  Integral Gain/1 -> Discrete-Time Integrator/1
  x/1 -> Derivative Gain/1, Integral Gain/1, Gain/1

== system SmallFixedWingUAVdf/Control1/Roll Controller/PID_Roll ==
  x : Inport
  reset_i : Inport  Port=2
  Derivative Gain : Gain  DisableCoverage=on  Gain=0  ParamMin=-100  ParamMax=100  OutMin=-100  OutMax=100
  Discrete Derivative : simulink/Discrete/Discrete Derivative  gainval=1.0  ICPrevScaledInput=0.0  OutMin=[]  OutMax=[]  OutDataType=fixdt(1, 16)  OutScaling=2^-10  DoSatur=off
  Discrete-Time Integrator : DiscreteIntegrator  ExternalReset=either  SampleTime=-1  ICPrevOutput=DiscIntNeverNeededParam  ICPrevScaledInput=DiscIntNeverNeededParam
  Gain : Gain  Gain=9
  Integral Gain : Gain  DisableCoverage=on  Gain=0.4
  Sum : Sum  Inputs=+++
  y : Outport  InitialOutput=0  VectorParamsAs1DForOutWhenUnconnected=off
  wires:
  reset_i/1 -> Discrete-Time Integrator/2
  Discrete-Time Integrator/1 -> Sum/2
  Discrete Derivative/1 -> Sum/3
  Sum/1 -> y/1
  Gain/1 -> Sum/1
  Derivative Gain/1 -> Discrete Derivative/1
  Integral Gain/1 -> Discrete-Time Integrator/1
  x/1 -> Derivative Gain/1, Integral Gain/1, Gain/1

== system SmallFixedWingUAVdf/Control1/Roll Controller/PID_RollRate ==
  x : Inport
  reset_i : Inport  Port=2
  Derivative Gain : Gain  DisableCoverage=on  Gain=0.01  ParamMin=-100  ParamMax=100  OutMin=-100  OutMax=100
  Discrete Derivative : simulink/Discrete/Discrete Derivative  gainval=1.0  ICPrevScaledInput=0.0  OutMin=[]  OutMax=[]  OutDataType=fixdt(1, 16)  OutScaling=2^-10  DoSatur=off
  Discrete-Time Integrator : DiscreteIntegrator  ExternalReset=either  SampleTime=-1  LimitOutput=on  UpperSaturationLimit=0.3  LowerSaturationLimit=-0.3  ICPrevOutput=DiscIntNeverNeededParam  ICPrevScaledInput=DiscIntNeverNeededParam
  Gain : Gain  Gain=0.8
  Integral Gain : Gain  DisableCoverage=on  Gain=2
  Sum : Sum  Inputs=+++
  y : Outport  InitialOutput=0  VectorParamsAs1DForOutWhenUnconnected=off
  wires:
  x/1 -> Gain/1, Integral Gain/1, Derivative Gain/1
  Integral Gain/1 -> Discrete-Time Integrator/1
  Derivative Gain/1 -> Discrete Derivative/1
  Gain/1 -> Sum/1
  Sum/1 -> y/1
  Discrete Derivative/1 -> Sum/3
  Discrete-Time Integrator/1 -> Sum/2
  reset_i/1 -> Discrete-Time Integrator/2

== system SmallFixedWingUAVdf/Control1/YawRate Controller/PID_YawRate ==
  x : Inport
  reset_i : Inport  Port=2
  Derivative Gain : Gain  DisableCoverage=on  Gain=0.3  ParamMin=-100  ParamMax=100  OutMin=-100  OutMax=100
  Discrete Derivative : simulink/Discrete/Discrete Derivative  gainval=1.0  ICPrevScaledInput=0.0  OutMin=[]  OutMax=[]  OutDataType=fixdt(1, 16)  OutScaling=2^-10  DoSatur=off
  Discrete-Time Integrator : DiscreteIntegrator  ExternalReset=either  SampleTime=-1  LimitOutput=on  UpperSaturationLimit=0.3  LowerSaturationLimit=-0.3  ICPrevOutput=DiscIntNeverNeededParam  ICPrevScaledInput=DiscIntNeverNeededParam
  Gain : Gain  Gain=4
  Integral Gain : Gain  DisableCoverage=on  Gain=3
  Sum : Sum  Inputs=+++
  y : Outport  InitialOutput=0  VectorParamsAs1DForOutWhenUnconnected=off
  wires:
  reset_i/1 -> Discrete-Time Integrator/2
  Discrete-Time Integrator/1 -> Sum/2
  Discrete Derivative/1 -> Sum/3
  Sum/1 -> y/1
  Gain/1 -> Sum/1
  Derivative Gain/1 -> Discrete Derivative/1
  Integral Gain/1 -> Discrete-Time Integrator/1
  x/1 -> Derivative Gain/1, Integral Gain/1, Gain/1

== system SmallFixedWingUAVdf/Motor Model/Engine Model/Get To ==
  dt : Inport
  Divide : Product  Inputs=3
  Math Function : Math  Operator=pow  SignedPower=on
  Math Function1 : Math  Operator=pow  SignedPower=on
  MaxRPM : Gain  Gain=7200  SaturateOnIntegerOverflow=on
  MaxRPM1 : Gain  Gain=uav.engine.TFact  SaturateOnIntegerOverflow=on
  Min RPM : Constant  Value=2000
  Min Th K : Constant  Value=uav.engine.MinThK
  Prop Diameter (in) : Constant  Value=17
  Prop Diameter (in)1 : Constant  Value=2
  Prop Diameter (in)2 : Constant  Value=4
  Saturation : Saturate  UpperLimit=1.0  LowerLimit=0
  Sum : Sum  Inputs=|++
  Sum1 : Sum  Inputs=|++
  Th K : Gain  Gain=uav.engine.ThK  SaturateOnIntegerOverflow=on
  To Constant : Constant  Value=2.83e-12
  To : Outport  VectorParamsAs1DForOutWhenUnconnected=off
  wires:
  Min Th K/1 -> Sum1/2
  Sum1/1 -> MaxRPM/1
  dt/1 -> Saturation/1
  Th K/1 -> Sum1/1
  MaxRPM/1 -> Sum/1
  Min RPM/1 -> Sum/2
  Sum/1 -> Math Function/1
  MaxRPM1/1 -> To/1
  Divide/1 -> MaxRPM1/1
  To Constant/1 -> Divide/3
  Math Function1/1 -> Divide/2
  Math Function/1 -> Divide/1
  Prop Diameter (in)/1 -> Math Function1/1
  Prop Diameter (in)2/1 -> Math Function1/2
  Prop Diameter (in)1/1 -> Math Function/2
  Saturation/1 -> Th K/1

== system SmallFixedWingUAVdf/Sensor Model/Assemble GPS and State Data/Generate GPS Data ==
  XYZ (NEU) : Inport
  Bus Creator : BusCreator  Inputs=2
  Flat Earth to LLA : aerolibtransform2/Flat Earth to LLA  units=Metric (MKS)  ptype=Earth (WGS84)  F=1/298.257223563  R=6378137  refPosPort=off  LL0=uav.ic.gsLL  psi=0
  Zero level trust : Constant  Value=0
  GPSData : Outport  VectorParamsAs1DForOutWhenUnconnected=off
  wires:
  Bus Creator/1 -> GPSData/1
  Flat Earth to LLA/1 -> Bus Creator/1  "gps_latLon"
  Zero level trust/1 -> Flat Earth to LLA/2
  XYZ (NEU)/1 -> Flat Earth to LLA/1
  Flat Earth to LLA/2 -> Bus Creator/2  "gps_h"

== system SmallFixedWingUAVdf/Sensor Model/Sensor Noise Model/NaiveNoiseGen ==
  Signal In : Inport
  Noise On : Inport  Port=2
  Add : Sum
  Band-Limited White Noise : simulink/Sources/Band-Limited White Noise  Cov=np  Ts=st  seed=ns
  Gain : Gain  Gain=ng
  Switch : Switch  Threshold=0.3
  Signal Out : Outport  VectorParamsAs1DForOutWhenUnconnected=off
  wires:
  Gain/1 -> Add/2
  Signal In/1 -> Add/1, Switch/3
  Switch/1 -> Signal Out/1
  Noise On/1 -> Switch/2
  Add/1 -> Switch/1
  Band-Limited White Noise/1 -> Gain/1

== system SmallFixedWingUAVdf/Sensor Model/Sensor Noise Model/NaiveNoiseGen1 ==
  Signal In : Inport
  Noise On : Inport  Port=2
  Add : Sum
  Band-Limited White Noise : simulink/Sources/Band-Limited White Noise  Cov=np  Ts=st  seed=ns
  Gain : Gain  Gain=ng
  Switch : Switch  Threshold=0.3
  Signal Out : Outport  VectorParamsAs1DForOutWhenUnconnected=off
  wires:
  Gain/1 -> Add/2
  Signal In/1 -> Add/1, Switch/3
  Switch/1 -> Signal Out/1
  Noise On/1 -> Switch/2
  Add/1 -> Switch/1
  Band-Limited White Noise/1 -> Gain/1

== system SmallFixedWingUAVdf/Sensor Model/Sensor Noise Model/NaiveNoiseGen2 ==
  Signal In : Inport
  Noise On : Inport  Port=2
  Add : Sum
  Band-Limited White Noise : simulink/Sources/Band-Limited White Noise  Cov=np  Ts=st  seed=ns
  Gain : Gain  Gain=ng
  Switch : Switch  Threshold=0.3
  Signal Out : Outport  VectorParamsAs1DForOutWhenUnconnected=off
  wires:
  Gain/1 -> Add/2
  Signal In/1 -> Add/1, Switch/3
  Switch/1 -> Signal Out/1
  Noise On/1 -> Switch/2
  Add/1 -> Switch/1
  Band-Limited White Noise/1 -> Gain/1

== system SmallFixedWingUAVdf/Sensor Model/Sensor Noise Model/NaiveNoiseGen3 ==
  Signal In : Inport
  Noise On : Inport  Port=2
  Add : Sum
  Band-Limited White Noise : simulink/Sources/Band-Limited White Noise  Cov=np  Ts=st  seed=ns
  Gain : Gain  Gain=ng
  Switch : Switch  Threshold=0.3
  Signal Out : Outport  VectorParamsAs1DForOutWhenUnconnected=off
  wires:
  Gain/1 -> Add/2
  Signal In/1 -> Add/1, Switch/3
  Switch/1 -> Signal Out/1
  Noise On/1 -> Switch/2
  Add/1 -> Switch/1
  Band-Limited White Noise/1 -> Gain/1

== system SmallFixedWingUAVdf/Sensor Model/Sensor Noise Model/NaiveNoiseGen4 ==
  Signal In : Inport
  Noise On : Inport  Port=2
  Add : Sum
  Band-Limited White Noise : simulink/Sources/Band-Limited White Noise  Cov=np  Ts=st  seed=ns
  Gain : Gain  Gain=ng
  Switch : Switch  Threshold=0.3
  Signal Out : Outport  VectorParamsAs1DForOutWhenUnconnected=off
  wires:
  Gain/1 -> Add/2
  Signal In/1 -> Add/1, Switch/3
  Switch/1 -> Signal Out/1
  Noise On/1 -> Switch/2
  Add/1 -> Switch/1
  Band-Limited White Noise/1 -> Gain/1

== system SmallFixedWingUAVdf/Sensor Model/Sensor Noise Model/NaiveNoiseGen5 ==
  Signal In : Inport
  Noise On : Inport  Port=2
  Add : Sum
  Band-Limited White Noise : simulink/Sources/Band-Limited White Noise  Cov=np  Ts=st  seed=ns
  Gain : Gain  Gain=ng
  Switch : Switch  Threshold=0.3
  Signal Out : Outport  VectorParamsAs1DForOutWhenUnconnected=off
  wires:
  Gain/1 -> Add/2
  Signal In/1 -> Add/1, Switch/3
  Switch/1 -> Signal Out/1
  Noise On/1 -> Switch/2
  Add/1 -> Switch/1
  Band-Limited White Noise/1 -> Gain/1

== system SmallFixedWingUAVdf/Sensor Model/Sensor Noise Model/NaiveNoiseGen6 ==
  Signal In : Inport
  Noise On : Inport  Port=2
  Add : Sum
  Band-Limited White Noise : simulink/Sources/Band-Limited White Noise  Cov=np  Ts=st  seed=ns
  Gain : Gain  Gain=ng
  Switch : Switch  Threshold=0.3
  Signal Out : Outport  VectorParamsAs1DForOutWhenUnconnected=off
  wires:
  Gain/1 -> Add/2
  Signal In/1 -> Add/1, Switch/3
  Switch/1 -> Signal Out/1
  Noise On/1 -> Switch/2
  Add/1 -> Switch/1
  Band-Limited White Noise/1 -> Gain/1

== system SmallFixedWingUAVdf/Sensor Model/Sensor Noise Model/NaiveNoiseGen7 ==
  Signal In : Inport
  Noise On : Inport  Port=2
  Add : Sum
  Band-Limited White Noise : simulink/Sources/Band-Limited White Noise  Cov=np  Ts=st  seed=ns
  Gain : Gain  Gain=ng
  Switch : Switch  Threshold=0.3
  Signal Out : Outport  VectorParamsAs1DForOutWhenUnconnected=off
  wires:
  Gain/1 -> Add/2
  Signal In/1 -> Add/1, Switch/3
  Switch/1 -> Signal Out/1
  Noise On/1 -> Switch/2
  Add/1 -> Switch/1
  Band-Limited White Noise/1 -> Gain/1

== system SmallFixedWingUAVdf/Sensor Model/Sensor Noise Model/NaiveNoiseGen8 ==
  Signal In : Inport
  Noise On : Inport  Port=2
  Add : Sum
  Band-Limited White Noise : simulink/Sources/Band-Limited White Noise  Cov=np  Ts=st  seed=ns
  Gain : Gain  Gain=ng
  Switch : Switch  Threshold=0.3
  Signal Out : Outport  VectorParamsAs1DForOutWhenUnconnected=off
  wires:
  Gain/1 -> Add/2
  Signal In/1 -> Add/1, Switch/3
  Switch/1 -> Signal Out/1
  Noise On/1 -> Switch/2
  Add/1 -> Switch/1
  Band-Limited White Noise/1 -> Gain/1

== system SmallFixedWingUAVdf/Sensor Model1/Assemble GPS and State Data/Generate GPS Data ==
  XYZ (NEU) : Inport
  Bus Creator : BusCreator  Inputs=2
  Flat Earth to LLA : aerolibtransform2/Flat Earth to LLA  units=Metric (MKS)  ptype=Earth (WGS84)  F=1/298.257223563  R=6378137  refPosPort=off  LL0=uav.ic.gsLL  psi=0
  Zero level trust : Constant  Value=0
  GPSData : Outport  VectorParamsAs1DForOutWhenUnconnected=off
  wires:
  Bus Creator/1 -> GPSData/1
  Flat Earth to LLA/1 -> Bus Creator/1  "gps_latLon"
  Zero level trust/1 -> Flat Earth to LLA/2
  XYZ (NEU)/1 -> Flat Earth to LLA/1
  Flat Earth to LLA/2 -> Bus Creator/2  "gps_h"

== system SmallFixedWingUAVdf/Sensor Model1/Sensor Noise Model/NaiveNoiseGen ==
  Signal In : Inport
  Noise On : Inport  Port=2
  Add : Sum
  Band-Limited White Noise : simulink/Sources/Band-Limited White Noise  Cov=np  Ts=st  seed=ns
  Gain : Gain  Gain=ng
  Switch : Switch  Threshold=0.3
  Signal Out : Outport  VectorParamsAs1DForOutWhenUnconnected=off
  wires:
  Gain/1 -> Add/2
  Signal In/1 -> Add/1, Switch/3
  Switch/1 -> Signal Out/1
  Noise On/1 -> Switch/2
  Add/1 -> Switch/1
  Band-Limited White Noise/1 -> Gain/1
